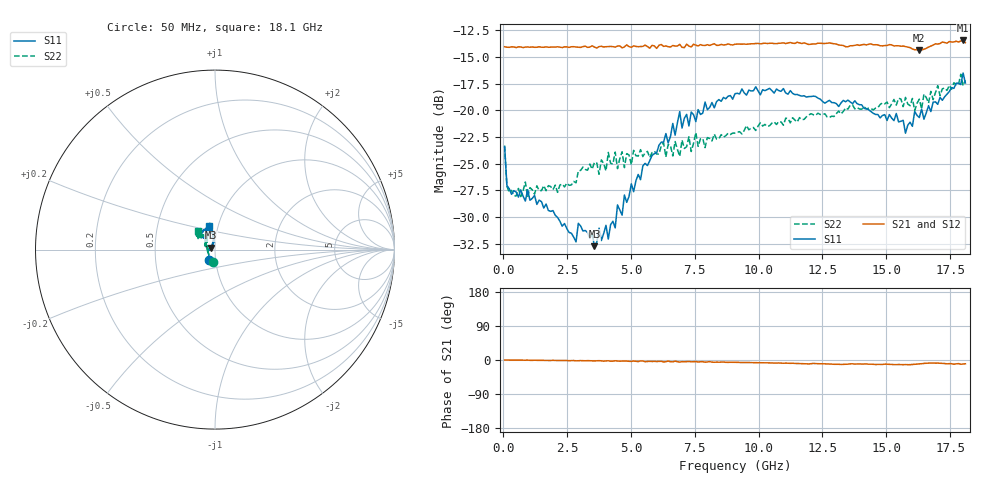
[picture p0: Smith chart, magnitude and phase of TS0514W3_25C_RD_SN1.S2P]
! Network Analyzer HP8720D.06.14 Serial No. US36140669
! 17 Jun 2005  08:24:18
! Frequency  S11  S21  S12  S22
# HZ  S  DB R 50
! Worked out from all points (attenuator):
!   201 points, 50 MHz to 18.1 GHz, reference 50 ohm
!   highest |S21| = -13.44 dB at 18.01 GHz (marker M1); lowest = -14.4 dB at 16.3 GHz (marker M2)
!   lowest |S11| = -32.7 dB at 3.57 GHz (marker M3), VSWR 1.05, Z = 48 + j1.05 ohm
!   |S11| at or under -10 dB: start of sweep to end of sweep
!   |S22| runs from -28.1 to -16.6 dB; largest |S21 - S12| = 0.0061
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5e7  -23.40 -117.7  -14.03 -0.2  -14.05 -0.0  -23.30 -97.8
1.4025e8  -27.03 -141.4  -14.07 -0.2  -14.06 -0.1  -27.11 -140.0
4.11e8  -27.52 -164.0  -14.05 -0.3  -14.06 -0.2  -27.99 -165.0
2.84775e9  -32.32 174.7  -14.05 -2.2  -14.06 -1.9  -26.78 150.0
2.938e9  -30.58 169.1  -14.07 -2.0  -14.02 -2.1  -25.68 162.5
3.1185e9  -31.30 164.8  -14.02 -1.9  -14.05 -2.0  -25.31 161.5
3.56975e9  -32.73 151.9  -14.06 -2.5  -14.08 -2.6  -24.86 155.4
4.11125e9  -32.06 126.8  -14.01 -2.1  -13.98 -2.7  -23.94 154.4
6.09675e9  -23.26 94.9  -13.89 -3.6  -13.85 -3.6  -24.09 144.2
6.7285e9  -22.32 99.2  -13.96 -3.0  -14.07 -3.9  -22.92 137.5
6.909e9  -20.11 97.5  -13.80 -5.5  -13.96 -4.8  -24.31 132.5
7.27e9  -21.45 94.8  -13.96 -3.9  -13.97 -5.0  -22.46 134.4
7.36025e9  -20.15 91.6  -14.05 -4.9  -13.96 -4.1  -23.85 137.3
7.54075e9  -21.05 93.1  -13.87 -4.0  -13.78 -5.4  -22.07 136.5
7.90175e9  -19.21 99.9  -13.91 -5.8  -13.88 -5.1  -23.48 129.3
9.075e9  -18.43 108.5  -13.79 -6.1  -13.79 -6.1  -22.12 124.7
1.21435e10  -18.66 133.8  -13.76 -9.0  -13.75 -9.2  -20.41 125.0
1.512175e10  -20.39 131.1  -13.83 -11.6  -13.79 -11.0  -19.74 136.2
1.57535e10  -22.13 127.7  -14.01 -12.0  -14.08 -12.5  -18.78 134.6
1.6295e10  -20.67 118.4  -14.36 -10.3  -14.27 -10.7  -18.94 144.5
1.800975e10  -16.48 101.1  -13.44 -10.7  -13.54 -10.3  -17.68 139.9
1.81e10  -17.43 103.3  -13.64 -10.0  -13.72 -11.5  -17.18 133.1
